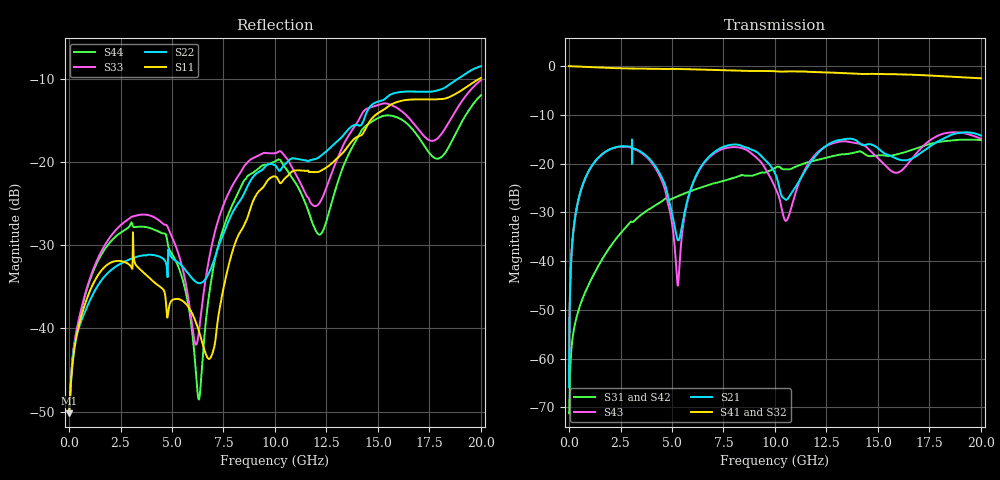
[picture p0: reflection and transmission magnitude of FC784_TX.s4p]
! Touchstone generated by fitter/viewer
# HZ S  RI R 5.000000e+001
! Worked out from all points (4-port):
!   4999 points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, 4.001 MHz to 20 GHz, reference 50 ohm
!   strongest paths, dB at 4.001 MHz, 5.001 GHz, 10 GHz, 15 GHz, 20 GHz:
!     S41: 0.0, -0.6, -1.1, -1.6, -2.5
!     S32: 0.0, -0.6, -1.1, -1.8, -2.9
!     S21: -65.8, -30.2, -22.0, -16.8, -14.3
!     S43: -65.8, -32.2, -24.9, -18.9, -14.9
!     S31: -71.2, -27.2, -20.9, -18.3, -15.2
!     S42: -71.2, -27.3, -21.0, -18.4, -15.4
!   lowest |S11| = -50.2 dB at 4.001 MHz (marker M1), VSWR 1.01, Z = 50.3 + j0.0208 ohm
!   |S11| at or under -10 dB: start of sweep to 19.94 GHz
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4000800  0.00309 0.000206  0.00027 0.000433  -0.000266 -7.15e-05  0.9969 -0.00287
         0.00027 0.000433  0.00309 0.000216  0.9969 -0.00289  -0.000266 -7.15e-05
         -0.000266 -7.15e-05  0.9969 -0.00289  0.00309 0.000218  0.00027 0.000433
         0.9969 -0.00287  -0.000266 -7.15e-05  0.00027 0.000433  0.00309 0.000208
1.512302e9  -0.00958 -0.0196  0.0952 0.0727  -0.00683 -0.0068  0.5746 -0.7739
            0.0952 0.0727  -0.00976 -0.0163  0.57 -0.7772  -0.00695 -0.00715
            -0.00683 -0.0068  0.57 -0.7772  0.00274 -0.028  0.0984 0.0679
            0.5746 -0.7739  -0.00695 -0.00715  0.0984 0.0679  -0.000101 -0.027
5.117023e9  0.0132 0.00707  0.0177 -0.0148  -0.00359 0.0445  -0.9321 -0.06
            0.0177 -0.0148  0.0191 0.0174  -0.9329 -0.0402  -0.00414 0.0445
            -0.00359 0.0445  -0.9329 -0.0402  -0.0321 0.00619  0.00529 -0.0142
            -0.9321 -0.06  -0.00414 0.0445  0.00529 -0.0142  -0.0264 -0.00216
6.309262e9  0.00909 -0.00312  0.0583 0.0626  0.0347 0.0439  -0.7316 0.56
            0.0583 0.0626  0.0157 0.0101  -0.7166 0.5787  0.0345 0.0444
            0.0347 0.0439  -0.7166 0.5787  0.00863 0.00422  0.0611 0.0577
            -0.7316 0.56  0.0345 0.0444  0.0611 0.0577  -0.00166 -0.00336
1.001e10  0.0807 -0.0134  0.0583 -0.053  0.0155 -0.089  0.8467 0.2545
          0.0583 -0.053  0.095 -0.00502  0.8552 0.2167  0.0118 -0.0885
          0.0155 -0.089  0.8552 0.2167  -0.0937 -0.0628  -0.0114 -0.0555
          0.8467 0.2545  0.0118 -0.0885  -0.0114 -0.0555  -0.0793 -0.0622
1.563113e10  0.177 -0.1318  0.098 -0.0684  0.0268 0.1175  -0.821 -0.0852
             0.098 -0.0684  0.2109 -0.142  -0.8123 -0.0297  0.0227 0.1182
             0.0268 0.1175  -0.8123 -0.0297  -0.1809 -0.1248  -0.0803 -0.0262
             -0.821 -0.0852  0.0227 0.1182  -0.0803 -0.0262  -0.1408 -0.127
2e10  0.159 -0.2768  0.0848 -0.1738  0.0108 -0.1737  0.5982 0.4501
      0.0848 -0.1738  0.1789 -0.3304  0.6187 0.3615  0.0133 -0.1702
      0.0108 -0.1737  0.6187 0.3615  0.0468 -0.306  0.00166 -0.1796
      0.5982 0.4501  0.0133 -0.1702  0.00166 -0.1796  0.0707 -0.241
